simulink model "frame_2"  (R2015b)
settings: Solver=ode45  StartTime=0.0  StopTime=40  RelTol=1e-3
undefined symbols (not defined in the file or in its folder): fir1
libraries: dspsigops x2, simulink x1, dspstat3 x1

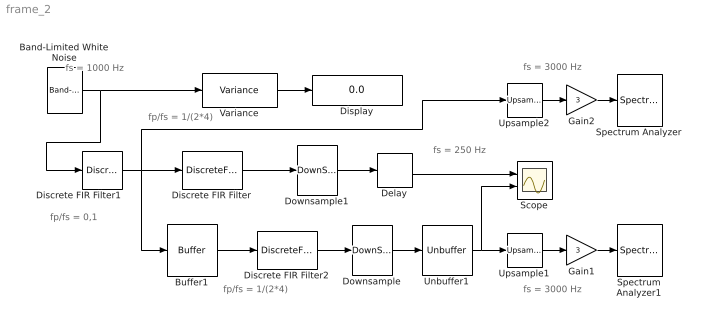
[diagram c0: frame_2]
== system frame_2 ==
  note: fs = 3000 Hz
  note: fs = 250 Hz
  note: fp/fs = 1/(2*4)
  note: fp/fs = 0,1
  note: fs = 1000 Hz
  note: fp/fs = 1/(2*4)
  note: fs = 3000 Hz
  Band-Limited White Noise : simulink/Sources/Band-Limited White Noise  Cov=1/1000  Ts=1/1000  seed=[23341]
  Buffer1 : Buffer  N=2048  TreatMby1Signals=One channel  OutputFrames=off
  Delay : Delay  DelayLength=2048*(1+1/4)
  Discrete FIR Filter : DiscreteFir  Coefficients=fir1(128, 0.25);
  Discrete FIR Filter1 : DiscreteFir  Coefficients=fir1(64, 0.2);
  Discrete FIR Filter2 : DiscreteFir  Coefficients=fir1(128, 0.25);  InputProcessing=Columns as channels (frame based)
  Display : Display
  Downsample : DownSample  N=4  RateOptions=Allow multirate processing
  Downsample1 : DownSample  N=4  RateOptions=Allow multirate processing
  Gain1 : Gain  Gain=3
  Gain2 : Gain  Gain=3
  Scope : Scope  NumInputPorts=2
  Spectrum Analyzer : SpectrumAnalyzer
  Spectrum Analyzer1 : SpectrumAnalyzer
  Unbuffer1 : Unbuffer  SampleBasedProcessing=Same as frame based
  Upsample1 : dspsigops/Upsample  N=3  phase=0  RateOptions=Allow multirate processing  ic=0  mode=Unused parameter value
  Upsample2 : dspsigops/Upsample  N=3  phase=0  RateOptions=Allow multirate processing  ic=0  mode=Unused parameter value
  Variance : dspstat3/Variance  run=on  reset_popup=None  directionMode=Each column  dimension=1  roiEnable=off  roiType=Rectangles  roiPortion=Entire ROI  roiOutput=Individual statistics for each ROI  roiFlag=off  roundingMode=Floor  overflowMode=off
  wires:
  Band-Limited White Noise/1 -> Variance/1, Discrete FIR Filter1/1
  Delay/1 -> Scope/1
  Variance/1 -> Display/1
  Buffer1/1 -> Discrete FIR Filter2/1
  Discrete FIR Filter2/1 -> Downsample/1
  Downsample/1 -> Unbuffer1/1
  Unbuffer1/1 -> Upsample1/1, Scope/2
  Discrete FIR Filter/1 -> Downsample1/1
  Downsample1/1 -> Delay/1
  Gain2/1 -> Spectrum Analyzer/1
  Upsample1/1 -> Gain1/1
  Gain1/1 -> Spectrum Analyzer1/1
  Discrete FIR Filter1/1 -> Upsample2/1, Discrete FIR Filter/1, Buffer1/1
  Upsample2/1 -> Gain2/1
